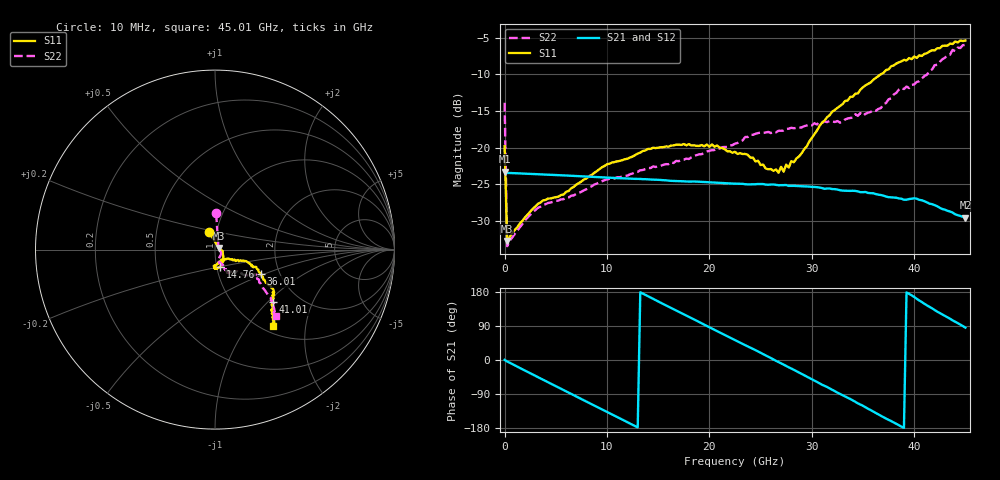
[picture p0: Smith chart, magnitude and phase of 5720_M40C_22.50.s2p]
! Device:  ADRF5720
! Description: 0.5dB LSB GaAs MMIC 6-bit Digital Attenuator
! Frequency:  0.000009 -  40 GHz
! Ports:
!	RF1	= Port 1
!	RF2	= Port 2
! Vdd:  3.3 Volt
! Vss:  -3.3 Volt
! Control:  0/3.3 Volt
! State:  22.50 dB attenuation
! Data:  The device was measured using G-S-G Probes on a matrix board.
!  Data was collected using an calibrated 4 port network analyzer.
!  The reference plane for this measurement is at the launchers.
! Note:  Analog Devices supplies this data as a sample of measured data
!  for this product.  Your particular data for this product may vary.
!  Data was taken at -40 degrees C.
!  Analog Devices reserves the right to change this data at anytime.
# GHZ S DB R 45.0
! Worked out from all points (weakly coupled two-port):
!   181 points, 10 MHz to 45.01 GHz, reference 45 ohm
!   highest |S21| = -23.26 dB at 10 MHz (marker M1); lowest = -29.5 dB at 45.01 GHz (marker M2)
!   lowest |S11| = -32.7 dB at 260 MHz (marker M3), VSWR 1.05, Z = 46.9 + j0.881 ohm
!   |S11| at or under -10 dB: start of sweep to 36.76 GHz
!   |S22| runs from -33.4 to -6.0 dB; largest |S21 - S12| = 0.00033
!   S11 on the Smith chart (normalised r, x): 10 MHz: 0.92, +0.18; 14.76 GHz: 1.04, -0.20; 36.01 GHz: 1.60, -0.47; 41.01 GHz: 1.49, -1.07; 45.01 GHz: 1.11, -1.34
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0.01  -19.82 108.8  -23.26 0.4  -23.28 0.4  -13.89 88.3
0.26  -32.73 24.0  -23.45 -3.8  -23.47 -3.8  -33.43 22.5
3.26  -27.67 -9.9  -23.63 -45.2  -23.65 -45.2  -28.20 -28.5
5.76  -26.40 -26.1  -23.78 -79.2  -23.81 -79.3  -27.03 -47.8
7.76  -24.34 -40.5  -23.92 -106.4  -23.94 -106.5  -25.81 -62.0
10.01  -22.28 -51.5  -24.09 -137.0  -24.11 -137.1  -24.34 -68.4
14.76  -20.06 -73.5  -24.38 158.1  -24.40 158.0  -22.64 -71.1
15.26  -19.94 -75.5  -24.41 151.1  -24.43 151.0  -22.48 -71.1
20.26  -19.57 -91.2  -24.75 83.0  -24.77 82.9  -20.36 -64.3
22.76  -20.86 -93.9  -24.92 49.3  -24.95 49.2  -19.37 -64.8
24.01  -21.37 -85.0  -25.01 32.7  -25.03 32.6  -18.25 -63.4
25.51  -22.85 -71.4  -25.04 11.6  -25.06 11.5  -17.95 -61.8
26.76  -23.42 -57.7  -25.13 -5.4  -25.15 -5.5  -17.70 -61.5
27.01  -22.62 -54.5  -25.12 -8.6  -25.14 -8.7  -17.71 -63.0
27.26  -23.28 -53.5  -25.11 -12.2  -25.13 -12.3  -17.68 -61.4
30.26  -18.18 -27.0  -25.36 -54.1  -25.39 -54.2  -16.68 -61.3
32.01  -15.10 -21.4  -25.65 -78.7  -25.67 -78.8  -16.45 -56.4
36.01  -10.76 -27.7  -26.22 -136.1  -26.25 -136.2  -14.88 -44.3
37.76  -8.91 -33.5  -26.78 -161.2  -26.81 -161.3  -13.29 -40.5
41.01  -7.22 -42.0  -27.31 148.2  -27.32 148.0  -10.25 -36.6
43.76  -5.88 -49.9  -28.85 104.6  -28.90 104.4  -6.69 -43.6
45.01  -5.41 -52.8  -29.54 85.3  -29.56 85.2  -6.00 -47.5
